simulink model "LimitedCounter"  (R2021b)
settings: Solver=FixedStepDiscrete  StartTime=0.0  StopTime=10.0  FixedStep=Auto  RelTol=1e-3  EnableMultiTasking=on

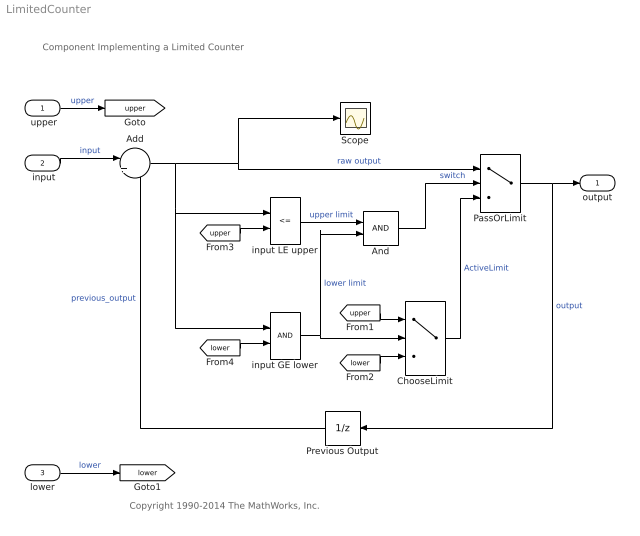
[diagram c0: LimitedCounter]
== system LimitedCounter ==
  note: Copyright 1990-2014 The MathWorks, Inc.
  note: Component Implementing a Limited Counter
  " upper" : Inport  OutDataTypeStr=double  PortDimensions=1
  " input" : Inport  Port=2  OutDataTypeStr=double  PortDimensions=1
  lower : Inport  Port=3  OutDataTypeStr=double  PortDimensions=1
  Add : Sum  Inputs=|++
  And : Logic  IconShape=distinctive
  ChooseLimit : Switch  Threshold=0.5
  PassOrLimit : Switch  Criteria=u2 ~= 0  Threshold=0.5
  Previous Output : UnitDelay  SampleTime=-1  HasFrameUpgradeWarning=on
  Scope : Scope
  input GE lower : RelationalOperator  Priority=1
  input LE upper : RelationalOperator  Priority=0  Operator=<=
  output : Outport  VectorParamsAs1DForOutWhenUnconnected=off
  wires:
  [upper] -> ChooseLimit/1
  PassOrLimit/1 -> output/1, Previous Output/1  "output"
  ChooseLimit/1 -> PassOrLimit/3  "ActiveLimit"
  input LE upper/1 -> And/1  "upper limit"
  Previous Output/1 -> Add/2  "previous_output"
  " input"/1 -> Add/1  "input"
  " upper"/1 -> [upper]  "upper"
  [lower] -> ChooseLimit/3
  [upper] -> input LE upper/2
  [lower] -> input GE lower/2
  input GE lower/1 -> And/2, ChooseLimit/2  "lower limit"
  lower/1 -> [lower]  "lower"
  And/1 -> PassOrLimit/2  "switch"
  Add/1 -> input GE lower/1, input LE upper/1, Scope/1, PassOrLimit/1  "raw output"
